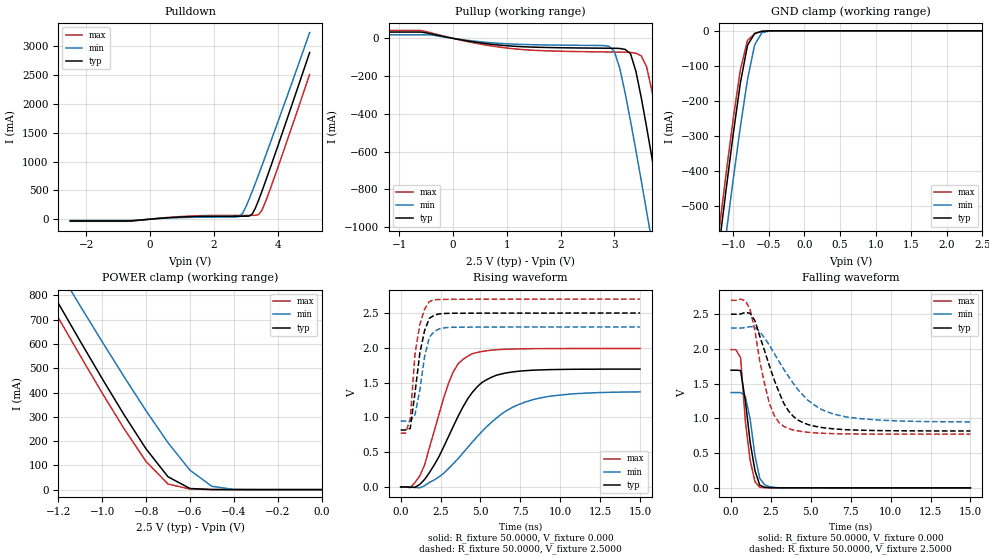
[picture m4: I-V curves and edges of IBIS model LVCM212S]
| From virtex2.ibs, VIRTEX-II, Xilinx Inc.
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|   Model LVCM212S
[Model]   LVCM212S
Model_type   I/O
Polarity   Non-Inverting
Enable   Active-Low
Vinh = 1.7V
Vinl = 0.7V
Vmeas =   1.2500V
Cref =  35.0000pF
Rref =   1.0000M
Vref =  0.000V
C_comp   7.0000pF   6.0000pF   8.0000pF
[Temperature Range]   25.0000   100.0000   0.000
[Voltage Range]   2.5000V   2.3000V   2.7000V
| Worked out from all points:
|   slope of the pulldown table from 0 to 0.375 V, typ, clamps not added: 21 ohm
|   slope of the pullup table from 0 to 0.375 V, typ, clamps not added: 20.5 ohm
|   GND clamp passes 1 mA (typ) near -0.57 V on its own axis
|   POWER clamp passes 1 mA (typ) near -0.52 V on its own axis
|   rising waveform, R_fixture 50.0000, V_fixture 0.000: 20-80 % time 2.32ns typ, 3.58ns min, 1.58ns max; typ from 0 V to 1.69 V
|   rising waveform, R_fixture 50.0000, V_fixture 2.5000: 20-80 % time 640ps typ, 615ps min, 528ps max; typ from 0.819 V to 2.5 V
|   falling waveform, R_fixture 50.0000, V_fixture 0.000: 20-80 % time 607ps typ, 576ps min, 505ps max; typ from 1.69 V to 0 V
|   falling waveform, R_fixture 50.0000, V_fixture 2.5000: 20-80 % time 1.64ns typ, 2.59ns min, 1.06ns max; typ from 2.5 V to 0.819 V
[Pulldown]
| voltage   I(typ)   I(min)   I(max)
-2.5V     -32.1mA    -21.59mA   -36.83mA
-700mV    -32.1mA    -21.59mA   -36.83mA
1.1V      40.81mA    29.55mA    49.66mA
2.8V      51.15mA    46.44mA    65.44mA
2.9V      51.24mA    103.4mA    65.54mA
3V        51.47mA    211.8mA    65.63mA
3.2V      87.52mA    480.7mA    65.92mA
3.4V      329.5mA    771.7mA    78.28mA
3.5V      477.3mA    920.6mA    151mA
3.7V      786.8mA    1.222A     424.4mA
4V        1.264A     1.68A      890.4mA
5V        2.892A     3.237A     2.511A
[Pullup]
| voltage   I(typ)   I(min)   I(max)
-2.5V     33.53mA    19.14mA    41.73mA
-600mV    33.53mA    19.14mA    41.73mA
1V        -38.92mA   -28.63mA   -51.11mA
2.9V      -52.1mA    -41.79mA   -72.07mA
3.1V      -53.39mA   -158.4mA   -72.65mA
3.3V      -81.13mA   -437.8mA   -74mA
3.5V      -314.2mA   -754.1mA   -92.11mA
3.6V      -471mA     -917.4mA   -151mA
3.8V      -802.6mA   -1.249A    -432.8mA
4V        -1.144A    -1.585A    -763.1mA
4.2V      -1.491A    -1.923A    -1.105A
5V        -2.897A    -3.292A    -2.506A
[GND_clamp]
| voltage   I(typ)   I(min)   I(max)
-2.5V     -2.881A    -2.936A    -2.838A
-1.2V     -617mA     -740.6mA   -570.6mA
-1.1V     -452.1mA   -579.7mA   -406.1mA
-1V       -293.4mA   -423mA     -249mA
-900mV    -148mA     -273.4mA   -110.1mA
-800mV    -41mA      -138.5mA   -27.22mA
-700mV    -7.569mA   -40.19mA   -8.128mA
-600mV    -1.403mA   -5.589mA   -1.597mA
-500mV    -127.6uA   -662.5uA   -122uA
2.5V      397.5nA    2.548uA    351.3nA
[POWER_clamp]
| voltage   I(typ)   I(min)   I(max)
-2.5V     2.874A     2.908A     2.816A
-1.3V     925.8mA    1.055A     866.1mA
-1.2V     767.5mA    905.5mA    707.7mA
-1.1V     610.9mA    756.3mA    551.2mA
-1V       456.9mA    609.1mA    397.6mA
-900mV    307.7mA    464.5mA    250.2mA
-800mV    167.5mA    324.6mA    115.6mA
-700mV    52.75mA    192.9mA    22.81mA
-600mV    4.571mA    79.88mA    2.444mA
-500mV    271.3uA    13.45mA    251.8uA
-400mV    16.93uA    820.9uA    15.04uA
0V        397.5nA    368nA      428.7nA
[Ramp]
| variable   typ   min   max
dV/dt_r   1.0164/2.3118n   0.8202/3.5760n   1.1940/1.6126n
dV/dt_f   1.0087/1.6280n   0.8105/2.5838n   1.1564/1.1102n
R_load = 50.0000
[Rising Waveform]
R_fixture = 50.0000
V_fixture = 0.000
| time   V(typ)   V(min)   V(max)
0s        6.981uV    8.2uV      6.729uV
600ps     -3.649mV   -137.9uV   -10.31mV
1.2ns     37.33mV    -12.94mV   159.6mV
2.1ns     315.3mV    100.7mV    800mV
3ns       725.2mV    264.2mV    1.49V
3.6ns     1.017V     407.9mV    1.771V
4.2ns     1.266V     568.3mV    1.879V
5.7ns     1.577V     932.1mV    1.966V
7.8ns     1.671V     1.22V      1.986V
15ns      1.694V     1.367V     1.99V
[Rising Waveform]
R_fixture = 50.0000
V_fixture = 2.5000
V_fixture_min = 2.3000
V_fixture_max = 2.7000
| time   V(typ)   V(min)   V(max)
0s        818.6mV    946.5mV    772.7mV
300ps     818.6mV    946.5mV    772.7mV
600ps     840.7mV    947.5mV    978.4mV
900ps     1.359V     1.041V     1.919V
1.2ns     1.922V     1.393V     2.335V
1.5ns     2.249V     1.875V     2.558V
1.8ns     2.425V     2.155V     2.666V
2.4ns     2.487V     2.272V     2.695V
3ns       2.495V     2.293V     2.697V
15ns      2.5V       2.299V     2.7V
[Falling Waveform]
R_fixture = 50.0000
V_fixture = 0.000
| time   V(typ)   V(min)   V(max)
0s        1.694V     1.372V     1.99V
300ps     1.694V     1.372V     1.99V
600ps     1.69V      1.373V     1.873V
900ps     1.244V     1.315V     948.5mV
1.2ns     651.6mV    983.7mV    391.5mV
1.5ns     246.5mV    462mV      88.56mV
1.8ns     38.27mV    136.8mV    7.769mV
2.1ns     9.096mV    45.79mV    2.659mV
3ns       1.209mV    1.233mV    1.14mV
15ns      -23.71uV   15.13uV    33.54uV
[Falling Waveform]
R_fixture = 50.0000
V_fixture = 2.5000
V_fixture_min = 2.3000
V_fixture_max = 2.7000
| time   V(typ)   V(min)   V(max)
0s        2.5V       2.3V       2.7V
900ps     2.526V     2.308V     2.695V
1.2ns     2.513V     2.322V     2.561V
1.5ns     2.404V     2.312V     2.256V
1.8ns     2.184V     2.247V     1.825V
2.4ns     1.759V     2.054V     1.217V
3.3ns     1.218V     1.708V     885.2mV
4.2ns     975.3mV    1.411V     820.3mV
6.3ns     852.2mV    1.071V     781.3mV
15ns      818.8mV    949.2mV    772.7mV
